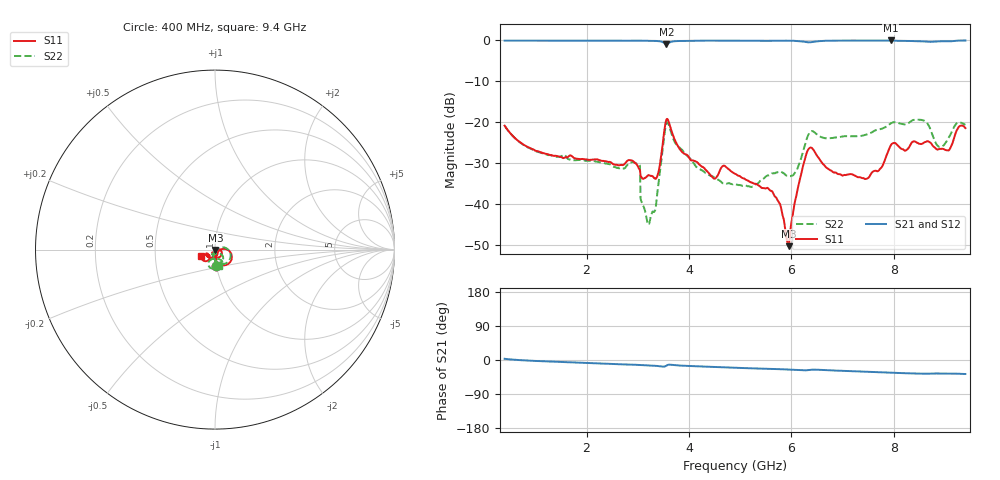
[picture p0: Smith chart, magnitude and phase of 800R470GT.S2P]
!  American Technical Ceramics  Date:  6/19/09
!  One Norden Lane
!  Huntington Station,  NY.  11746-2102
!  Tel:  (631) 622-4700  Fax:  (631) 622-4748
!  Part Number  800R470GT
!  Description: Ultra-low ESR, NPO  Mounting Orientation: Vertical
!  Application: High RF power Filters, Combiners, Matching networks,
!  Antenna, DC block, Bypass and Couplers
# GHZ S DB R 50
! Freq  |S11|  S11 Ph  |S21|  S21 Ph  |S12|  S12 Ph  |S22|  S22 Ph
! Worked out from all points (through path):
!   801 points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, 400 MHz to 9.4 GHz, reference 50 ohm
!   highest |S21| = 0.00 dB at 7.938 GHz (marker M1); lowest = -0.9 dB at 3.561 GHz (marker M2)
!   group delay of S21, straight-line fit = 11.9 ps
!   lowest |S11| = -50.4 dB at 5.946 GHz (marker M3), VSWR 1.01, Z = 50.3 - j0.16 ohm
!   |S11| at or under -10 dB: start of sweep to end of sweep
!   |S22| runs from -45.0 to -19.4 dB; largest |S21 - S12| = 0.0053
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0.4  -20.86 -85.8  -0.04 3.1  -0.07 3.2  -20.87 -86.0
0.996  -27.00 -88.9  -0.02 -2.5  -0.05 -2.4  -27.07 -92.9
1.908  -29.03 -85.9  -0.03 -7.5  -0.06 -7.4  -29.25 -103.0
2.999  -30.72 -75.8  -0.04 -12.9  -0.06 -12.8  -30.22 -125.4
3.1  -33.89 -66.2  -0.05 -13.6  -0.07 -13.5  -40.39 -102.5
3.201  -33.04 -52.1  -0.09 -14.3  -0.11 -14.2  -45.04 -68.1
3.325  -33.75 -38.9  -0.11 -15.0  -0.13 -14.9  -41.92 -17.5
3.404  -32.32 -9.9  -0.16 -16.0  -0.18 -15.9  -35.21 20.4
3.561  -19.37 -31.2  -0.92 -14.8  -0.94 -14.7  -20.19 -28.4
4.461  -33.50 -74.8  -0.03 -18.2  -0.05 -18.1  -33.28 -115.1
4.9  -32.66 -74.3  -0.06 -20.5  -0.07 -20.4  -35.16 -103.9
5.62  -36.91 -78.7  -0.09 -23.6  -0.10 -23.4  -32.58 -78.5
5.946  -50.38 -31.8  -0.06 -25.3  -0.07 -25.1  -33.26 -72.9
6.25  -29.75 -8.6  -0.31 -27.4  -0.31 -27.2  -26.31 -37.4
6.408  -26.40 -67.7  -0.38 -25.6  -0.38 -25.4  -22.19 -68.3
6.79  -31.95 -119.3  -0.06 -27.5  -0.05 -27.3  -23.91 -86.5
7.443  -33.94 -128.0  -0.01 -30.7  -0.01 -30.5  -23.11 -84.2
7.904  -26.73 -110.3  -0.01 -33.6  -0.01 -33.4  -20.65 -82.0
7.938  -25.79 -115.3  0.00 -33.8  -0.01 -33.6  -20.33 -83.4
8.59  -25.04 -145.3  -0.24 -36.2  -0.22 -36.0  -19.62 -104.5
8.905  -26.55 -146.6  -0.21 -35.9  -0.19 -35.6  -26.10 -89.0
9.4  -21.45 -156.9  -0.01 -36.9  -0.01 -36.6  -20.67 -75.9
